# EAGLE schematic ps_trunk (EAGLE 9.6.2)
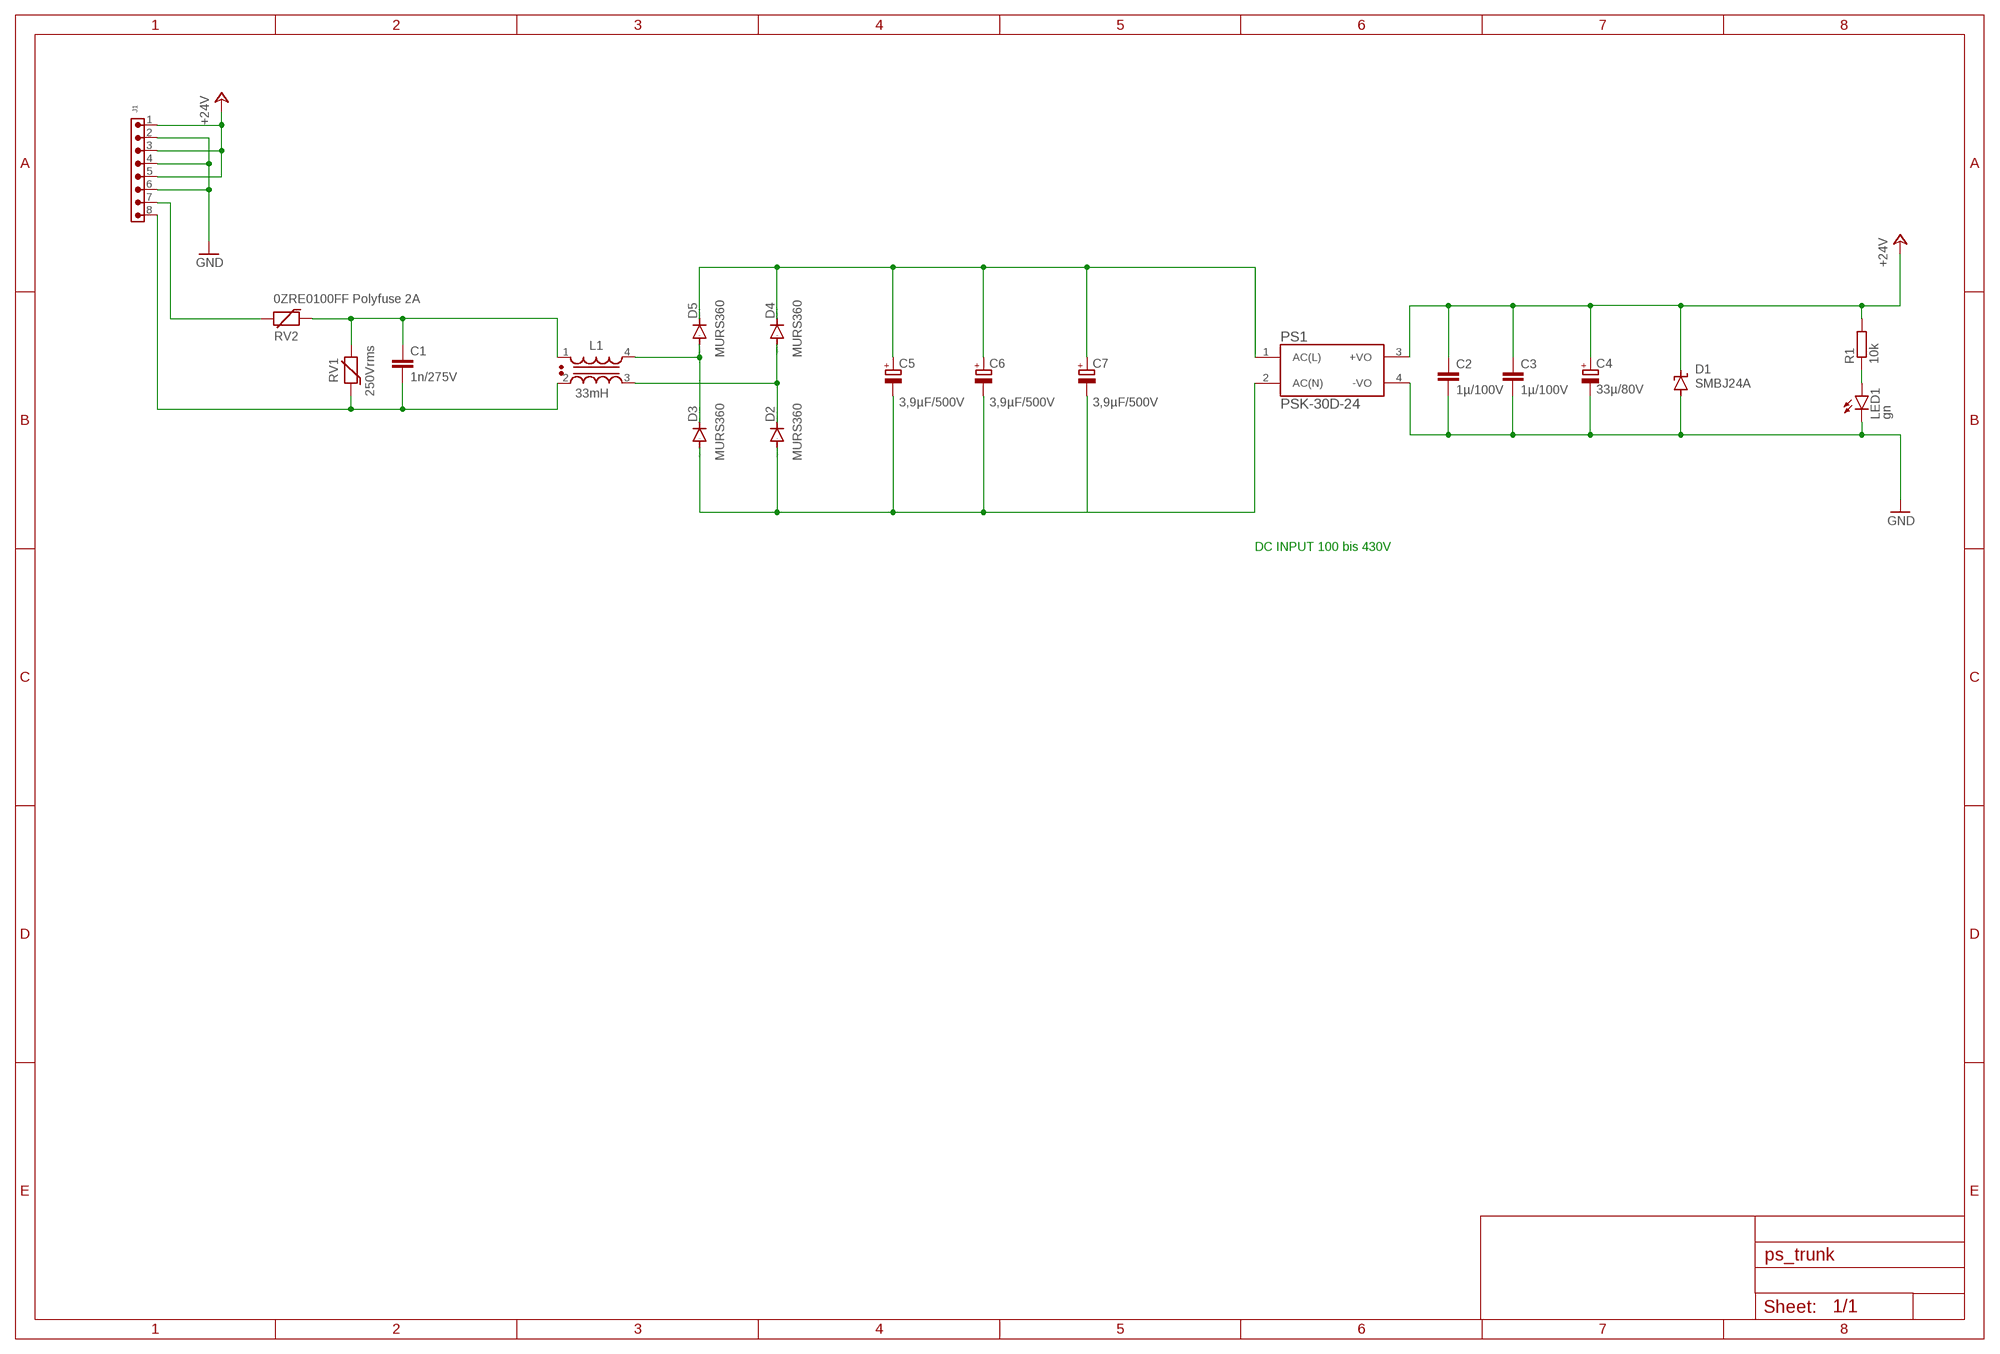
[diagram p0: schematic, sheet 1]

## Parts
C1  1n/275V  C-EU150-054X183  [C150-054X183]
C2  1µ/100V  C-EUC1210  [C1210]
C3  1µ/100V  C-EUC1210  [C1210]
C4  33µ/80V  CPOL-EUG  [PANASONIC_G]
C5  3,9µF/500V  CPOL-EUG  [PANASONIC_G]
C6  3,9µF/500V  CPOL-EUG  [PANASONIC_G]
C7  3,9µF/500V  CPOL-EUG  [PANASONIC_G]
D1  SMBJ24A  SUPPRESSOR-SMBJ  [SMBJ]
D2  MURS360  DIODE-SMC  [SMC]
D3  MURS360  DIODE-SMC  [SMC]
D4  MURS360  DIODE-SMC  [SMC]
D5  MURS360  DIODE-SMC  [SMC]
J1  691382000008  [691382000008]
L1  33mH  WE-CMBNC_M_7448030333  [WE-CMBNC_M_7448030333]
LED1  gn  LEDCHIP-LED0603  [CHIP-LED0603]
PS1  PSK-30D-24  [CONV_PSK-30D-24]
R1  10k  R-EU_R0603  [R0603]
RV1  250Vrms  WE-VD_20MM_820522511  [WE-VD_20MM_820522511]
RV2  0ZRE0100FF Polyfuse 2A  WE-VD_20MM_820422711  [WE-VD_20MM_820422711]

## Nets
+24V: C2.1 C3.1 C4.+ D1.C J1.1 J1.3 J1.5 PS1.3(+VO) R1.2
GND: C2.2 C3.2 C4.- D1.A J1.2 J1.4 J1.6 LED1.C PS1.4(-VO)
N$1: J1.7 RV2.2
N$2: C1.2 J1.8 L1.2 RV1.1
N$3: C1.1 L1.1 RV1.2 RV2.1
N$4: LED1.A R1.1
N$5: D3.C D5.A L1.4
N$6: D2.C D4.A L1.3
N$8: C5.+ C6.+ C7.+ D4.C D5.C PS1.1(AC(L))
N$9: C5.- C6.- C7.- D2.A D3.A PS1.2(AC(N))

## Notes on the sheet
- DC INPUT 100 bis 430V

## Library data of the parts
C1-C3 = rcl:C-EU: CAPACITOR, European symbol; SPICEPREFIX: C
C4-C7 = rcl:CPOL-EU: POLARIZED CAPACITOR, European symbol; SPICEPREFIX: C
D1 = diode:SUPPRESSOR-: Suppressor diode
D2-D5 = diode:DIODE-: DIODE
J1 = Wurth_Connectors_WR-TBL Pluggable Connector:691382000008: WR-TBL Serie 382 - 2.50 mm Vertical PCB Header KIND PROPERTIES Pitch 2.5 mm MATERIAL PROPERTIES Insulator Material PA66 Insulator Flammability Rating UL94 V-0 Contact Material Copper Alloy Contact Plating Tin Contact Type Stamped GENERAL INFORMATION Operating Temperature -40 up to +105 °C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; DATASHEET-URL: https://www.we-online.com/catalog/datasheet/691382000008.pdf; IR-UL: 12A; MOUNT: THT; PART-NUMBER: 691382000008; PINS: 8; PITCH: 2.5mm; TYPE: Vertical; WORKING-VOLTAGE-UL: 300V (AC)
L1 = Wurth_EMC Components_WE-CMBNC:WE-CMBNC_M: WE-CMBNC Common Mode Power Line Choke Nanocrystalline Characteristics Very high permeability nanocrystalline core material Improved isolation through plastic case and winding spacer High and stable inductance values up to 150 °C High rated currents Broadband suppression Small size Frequency range: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; DATASHEET-URL: https://www.we-online.com/catalog/datasheet/7448030333.pdf; IR: 2.5A; MOUNT: THT; PART-NUMBER: 7448030333; RDC: 90mOhm; VR: 250 V (AC); VT: 1500 V (AC)
LED1 = led:LED: LED
PS1 = PSK-30D-24:PSK-30D-24: 30 W, 85 - 305 Vac Input, Single Output, Encapsulated, Board Mount Ac-Dc Power Supply; MANUFACTURER: CUI Inc; MAXIMUM_PACKAGE_HEIGHT: 24.00mm; PARTREV: 1.0; STANDARD: Manufacturer Recommendations
R1 = rcl:R-EU_: RESISTOR, European symbol; SPICEPREFIX: R
RV1 = Wurth_EMC Components_WE-VD:WE-VD_20MM: WE-VD Disk Varistor; DATASHEET-URL: https://www.we-online.com/catalog/datasheet/820522511.pdf; ICLAMP: 100A; IPEAK: 6500A; MOUNT: THT; PART-NUMBER: 820522511; PDISS: 1W; VBR: 390V; VDC: 320Vdc; WMAX: 240J
RV2 = Wurth_EMC Components_WE-VD:WE-VD_20MM: WE-VD Disk Varistor; DATASHEET-URL: https://www.we-online.com/catalog/datasheet/820422711.pdf; ICLAMP: 100A; IPEAK: 10000A; MOUNT: THT; PART-NUMBER: 820422711; PDISS: 1W; VALUE: 275Vrms; VBR: 430V; VDC: 350Vdc; WMAX: 303J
